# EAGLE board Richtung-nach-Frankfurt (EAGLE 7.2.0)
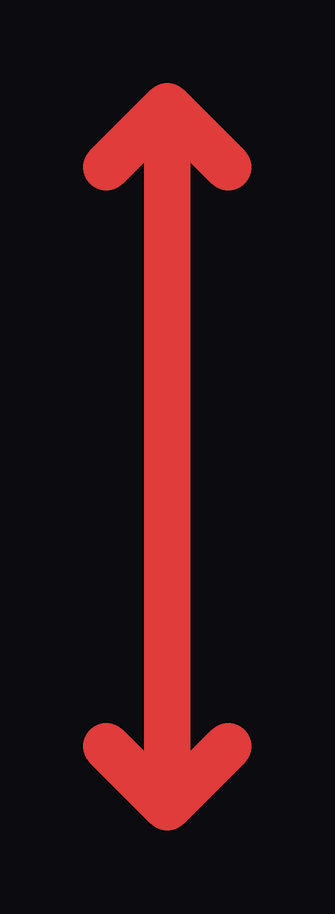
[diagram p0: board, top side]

No outline drawn. Coordinates in mm, seen from the top.
Copper layers (1*16): Top 0.035mm / dielectric 1.5mm / Bottom 0.035mm
Design rules "default": minimum track width 10mil, minimum drill 24mil, track to track 8mil, track to pad 8mil, pad to pad 8mil, via to via 8mil, smd to smd 8mil, copper to edge 40mil, drill to drill 8mil, minimum pad ring 10mil, minimum via ring 8mil, stop-mask expansion 4mil, vias tented up to drill 0mil, thermal gap 10mil

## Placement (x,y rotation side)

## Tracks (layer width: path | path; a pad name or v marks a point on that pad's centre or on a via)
S$1
  Top 1.93: 4.13,32.07 4.13,2.86 | 4.13,32.07 1.59,29.53 | 4.13,32.07 6.67,29.53 | 4.13,2.86 1.59,5.4 | 4.13,2.86 6.67,5.4

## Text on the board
tOrigins: Nach Frankfurt ausrichten !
